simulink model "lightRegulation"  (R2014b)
settings: Solver=ode3  StartTime=0.0  StopTime=inf  FixedStep=0.02  RelTol=1e-3
libraries: simulink x1, realtime_pacer_lib x1

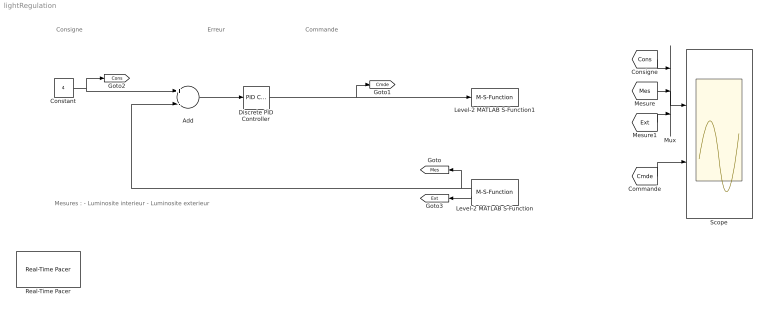
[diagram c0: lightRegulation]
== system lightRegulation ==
  note: Commande
  note: Mesures : - Luminosite interieur - Luminosite exterieur
  note: Consigne
  note: Erreur
  Add : Sum  Inputs=+-
  Constant : Constant  Value=4
  Discrete PID Controller : simulink/Continuous/PID Controller  Controller=I  TimeDomain=Discrete-time  SampleTime=0.02  IntegratorMethod=Forward Euler  FilterMethod=Forward Euler  Form=Parallel  P=0  I=6  D=0.05  N=100  InitialConditionSource=internal  InitialConditionForIntegrator=0  InitialConditionForFilter=0  ExternalReset=none  LimitOutput=on  UpperSaturationLimit=10  LowerSaturationLimit=0  LinearizeAsGain=off  AntiWindupMode=back-calculation  Kb=9  TrackingMode=off  Kt=1  PParamMin=[]  PParamMax=[]  IParamMin=[]  IParamMax=[]  DParamMin=[]  DParamMax=[]  NParamMin=[]  NParamMax=[]  KbParamMin=[]  KbParamMax=[]  KtParamMin=[]  KtParamMax=[]  POutMin=[]  POutMax=[]  IOutMin=[]  IOutMax=[]  DOutMin=[]  DOutMax=[]  NOutMin=[]  NOutMax=[]  KbOutMin=[]  KbOutMax=[]  KtOutMin=[]  KtOutMax=[]  IntegratorOutMin=[]  IntegratorOutMax=[]  FilterOutMin=[]  FilterOutMax=[]  SumOutMin=[]  SumOutMax=[]  SumI1OutMin=[]  SumI1OutMax=[]  SumI2OutMin=[]  SumI2OutMax=[]  SumI3OutMin=[]  SumI3OutMax=[]  SumDOutMin=[]  SumDOutMax=[]  SaturationOutMin=[]  SaturationOutMax=[]  IntegratorContinuousStateAttributes=''  IntegratorStateMustResolveToSignalObject=off  IntegratorRTWStateStorageClass=Auto  FilterContinuousStateAttributes=''  FilterStateMustResolveToSignalObject=off  FilterRTWStateStorageClass=Auto  DifferentiatorICPrevScaledInput=0  DifferentiatorOutMin=[]  DifferentiatorOutMax=[]  UseFilter=on
  Level-2 MATLAB S-Function : M-S-Function  FunctionName=analog_read
  Level-2 MATLAB S-Function1 : M-S-Function  FunctionName=analog_write
  Mux : Mux  Inputs=3
  Real-Time Pacer : realtime_pacer_lib/Real-Time Pacer  simTimePerRealTime=1
  Scope : Scope  NumInputPorts=2
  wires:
  [Cons] -> Mux/1
  [Mes] -> Mux/2
  Mux/1 -> Scope/1
  [Cmde] -> Scope/2
  Constant/1 -> Add/1, [Cons]
  Level-2 MATLAB S-Function/2 -> [Ext]
  [Ext] -> Mux/3
  Level-2 MATLAB S-Function/1 -> Add/2, [Mes]
  Add/1 -> Discrete PID Controller/1
  Discrete PID Controller/1 -> [Cmde], Level-2 MATLAB S-Function1/1
